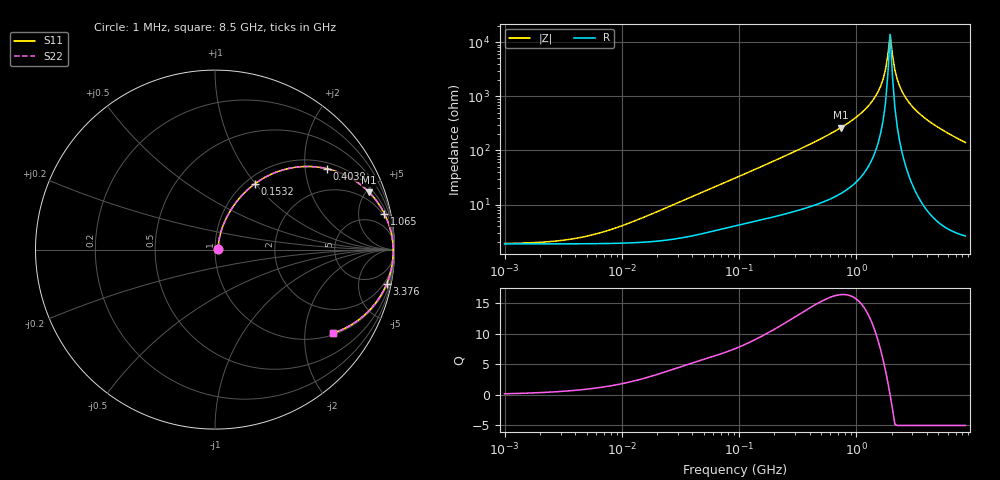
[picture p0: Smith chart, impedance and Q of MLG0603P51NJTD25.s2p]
! S-Parameter Data Generated by TDK Corporation
! Copyright(C) 2025 TDK Corporation.
! All Rights Reserved.
! TDK P/N: MLG0603P51NJTD25 (SMD / SMT Inductor (Coil))
! Property: L=51nH at 300MHz
! Size(LxWxT): 0.6x0.3x0.3mm
! Model Type: s2p (Touchstone File Format Version 1.0)
! Frequency: DC=Yes Start=1MHz Stop=8500MHz 198points Log-sweep
! Model Generated on Feb. 6, 2025
! Terms and conditions regarding TDK Simulation Models:
! 1)This simulation model is being provided solely for informational
!  purposes. Please refer to the specifications of the products in
!  terms of detailed characteristics of such products.
! 2)In no event shall TDK Corporation of any of its subsidiaries be
!  liable for any loss or damage arising, directly or indirectly,
!  from any information contained in this simulation model, including,
!  but not limited to loss or damages arising from any inaccuracies,
!  omissions or errors in connection with such information.
! 3)Any and all copyrights on this simulation model are owned by
!  TDK Corporation.  Duplication or redistribution of this simulation
!  model without prior written permission from TDK Corporation
!  is prohibited.
! 4)This simulation model is subject to any modification or change
!  without any prior notice.
! 5)Neither TDK Corporation nor any of its subsidiaries shall make any
!  warranty, express or implied, including but not limited to the
!  correctness, implied warranties of merchantability and fitness for
!  a particular purpose with respect to this simulation models.
! 6)The use of this simulation model shall be deemed to have consented
!  to the terms and conditions hereof.
! Port Assignments:
!  1 ---@@@--- 2
! Applicable Conditions:
!  Temperature = 25 degC
!  DC Bias Current = 0 A
!  Small Signal Operation
# Hz S MA R 50
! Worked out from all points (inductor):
!   197 points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, 1 MHz to 8.5 GHz, reference 50 ohm
!   read as one part in series: L = 56.2 nH near 17.5 MHz
!   highest Q = 16.4 at 736 MHz (marker M1), where L = 56.7 nH
!   self-resonance near 1.853 GHz
!   S11 on the Smith chart (normalised r, x): 1 MHz: 1.04, +0.01; 153.2 MHz: 1.10, +0.99; 403.9 MHz: 1.18, +2.62; 1.065 GHz: 1.61, +9.22; 3.376 GHz: 1, -10; 8.5 GHz: 1.05, -2.80
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1000000  0.01869 10.6  0.9816 -0.2  0.9816 -0.2  0.01869 10.6
4587603  0.02448 40.1  0.9814 -0.9  0.9814 -0.9  0.02448 40.1
8755050  0.0359 56.7  0.9807 -1.8  0.9807 -1.8  0.0359 56.7
2.10461e7  0.07554 69.9  0.9766 -4.2  0.9766 -4.2  0.07554 69.9
9.219544e7  0.284 66.1  0.9224 -16.4  0.9224 -16.4  0.284 66.1
1.531927e8  0.4285 58.8  0.8601 -25.2  0.8601 -25.2  0.4285 58.8
4.038753e8  0.7696 35.9  0.5871 -50.2  0.5871 -50.2  0.7696 35.9
4.229561e8  0.784 34.6  0.5694 -51.5  0.5694 -51.5  0.784 34.6
7.359901e8  0.9163 20.4  0.3488 -66.1  0.3488 -66.1  0.9163 20.4
1.064771e9  0.9644 12.0  0.2087 -74.2  0.2087 -74.2  0.9644 12.0
1.34121e9  0.9816 7.2  0.1265 -78.0  0.1265 -78.0  0.9816 7.2
1.613203e9  0.9895 3.6  0.06316 -78.6  0.06316 -78.6  0.9895 3.6
1.769233e9  0.9917 1.8  0.03214 -74.2  0.03214 -74.2  0.9917 1.8
1.852819e9  0.9924 0.9  0.01721 -63.5  0.01721 -63.5  0.9924 0.9
1.940355e9  0.9929 -0.0  0.007143 1.2  0.007143 1.2  0.9929 -0.0
2.032026e9  0.993 -0.9  0.01726 65.7  0.01726 65.7  0.993 -0.9
2.128028e9  0.9929 -1.8  0.03226 76.4  0.03226 76.4  0.9929 -1.8
2.333852e9  0.9918 -3.6  0.06356 80.8  0.06356 80.8  0.9918 -3.6
2.680511e9  0.9881 -6.4  0.1117 80.7  0.1117 80.7  0.9881 -6.4
3.37643e9  0.9754 -11.3  0.1955 77.2  0.1955 77.2  0.9754 -11.3
5.115526e9  0.9267 -21.1  0.36 67.9  0.36 67.9  0.9267 -21.1
8.5e9  0.8062 -35.2  0.5768 53.7  0.5768 53.7  0.8062 -35.2
